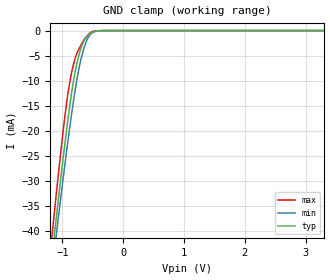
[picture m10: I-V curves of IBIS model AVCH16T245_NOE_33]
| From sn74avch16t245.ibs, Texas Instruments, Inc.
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[Model]   AVCH16T245_NOE_33
Model_type  Input
Vinl=0.8
Vinh=2.0
| variable   typ   min   max
C_comp   2.77pF   2.12pF   3.49pF
[Temperature Range]   40   100   -40
| Ambient temperature   25   85   -40
[Voltage range]   3.3   3   3.6
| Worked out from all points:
|   GND clamp passes 1 mA (typ) near -0.58 V on its own axis
[GND Clamp]
| AVCH16T245_NOE_33
|   Voltage   I(typ)   I(min)   I(max)
-4.6V     -463.5mA   -440.8mA   -490.1mA
-1.19V    -47.11mA   -49.96mA   -43.16mA
-1.16V    -43.79mA   -46.85mA   -39.57mA
-1.13V    -40.5mA    -43.76mA   -36.02mA
-1.105V   -37.79mA   -41.2mA    -33.1mA
-1.08V    -35.1mA    -38.66mA   -30.2mA
-950mV    -21.65mA   -25.86mA   -16.19mA
-835mV    -11.32mA   -15.45mA   -7.603mA
-760mV    -6.442mA   -9.645mA   -4.497mA
-670mV    -2.716mA   -4.542mA   -2.364mA
-500mV    -331.9uA   -373.2uA   -186.9uA
3.3V      251.3pA    1.067nA    59.37pA
